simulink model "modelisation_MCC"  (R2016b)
settings: Solver=ode15s  StartTime=0.0  StopTime=25  RelTol=1e-3  EnableMultiTasking=on
undefined symbols (not defined in the file): masse
libraries: fl_lib x13, bibliotheque_pilote x4, nesl_utility x2, elec_lib x1

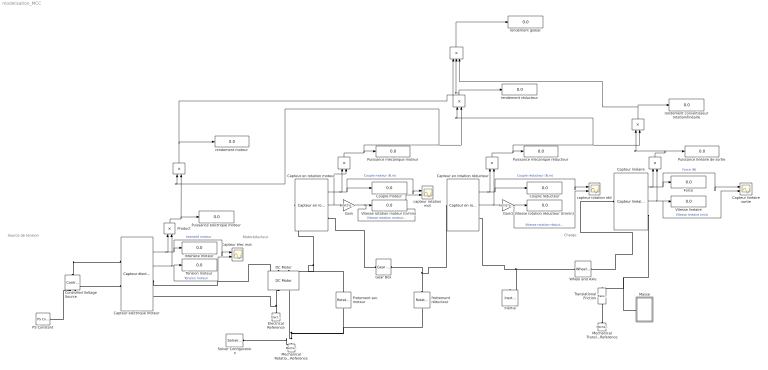
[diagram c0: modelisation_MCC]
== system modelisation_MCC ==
  note: Source de tension
  note: Motoréducteur
  note: Charge
  " " : Product
  " " : Product
  " " : Product
  "                          " : Product  Inputs=*/
  "                           " : Product  Inputs=*/
  "                              " : Product  Inputs=*/
  " " : Product  Inputs=3
  Capteur en rotation moteur : bibliotheque_pilote/Capteur en rotation
  Capteur en rotation réducteur : bibliotheque_pilote/Capteur en rotation
  Capteur linéaire : bibliotheque_pilote/Capteur linéaire
  Capteur linéaire sortie : Scope  NumInputPorts=2
  "Capteur élec mot " : Scope  NumInputPorts=2
  Capteur électrique moteur : bibliotheque_pilote/Capteur électrique
  Controlled Voltage Source : fl_lib/Electrical/Electrical Sources/Controlled Voltage Source
  Couple moteur : Display
  Couple réducteur : Display
  DC Motor : elec_lib/Actuators & Drivers/Rotational Actuators/DC Motor  parameterization=1  Ra=1.27 Ohm  La=0.17 H  emf_or_torque=2  Kv=0.00306 V/rpm  Ki=0.2188 N*m/A  T_stall=219 mN*m  w_max=3920 rpm  w_rated=2670 rpm  P_rated=20 W  V_rated=12 V  J=0.612 g*cm^2  lam_param=2  lam=0 N*m/(rad/s)  i_noload=290 mA  V_i_noload=12 V  speed0=0 rpm  alpha=0.00393 1/K  Tmeas=25 C  thermal_mass=100 J/K  initial_temperature=25 C
  Electrical Reference : fl_lib/Electrical/Electrical Elements/Electrical Reference
  Force : Display
  Frotement sec moteur : fl_lib/Mechanical/Rotational Elements/Rotational Friction  brkwy_trq=0.628 N*m  Col_trq=0.628 N*m  visc_coef=0 N*m/(rad/s)  trans_coef=10 s/rad  vel_thr=1e-04 rad/s  w_specify=off  w_priority=None  w=0 rad/s  t_specify=off  t_priority=None  t=0 N*m
  Gain : Gain  Gain=60/(2*pi)
  Gain1 : Gain  Gain=60/(2*pi)
  Gear Box : fl_lib/Mechanical/Mechanisms/Gear Box  ratio=18  t_in_specify=off  t_in_priority=High  t_in=0 N*m  t_out_specify=off  t_out_priority=High  t_out=0 N*m
  Inertia : fl_lib/Mechanical/Rotational Elements/Inertia  inertia=0.1512 g*cm^2  w_specify=off  w_priority=High  w=0 rad/s  t_specify=off  t_priority=High  t=0 N*m
  Intensité moteur : Display
  Masse : Subsystem
  Mechanical Rotational Reference : fl_lib/Mechanical/Rotational Elements/Mechanical Rotational Reference
  Mechanical Translational Reference : fl_lib/Mechanical/Translational Elements/Mechanical Translational Reference
  PS Constant : fl_lib/Physical Signals/Sources/PS Constant  constant=12
  Product : Product
  Puissance linéaire de sortie : Display
  Puissance mécanique moteur : Display
  Puissance mécanique réducteur : Display
  Puissance électrique moteur : Display
  Solver Configuration : nesl_utility/Solver Configuration  PhysicalDomain=network_engine_domain  SubClassName=solver  LeftPortType=input  RightPortType=generic  Accelerate=off  Tones=[]  Harmonics=[]  SimulateNoise=off  Profile=off  UseLocalSampling=off  EnableSwitchedLinearOptims=on  FrequencyDomain=off  UseCCode=off  RelTol=0.001  AbsTol=1e-06  MinStep=1e-09  ToWorkspace=off  RevertToSquareIcSolve=off  NumHomotopyIterations=100  PhasorMode=off  PhasorModeNumHarmonics=1  OverrideAbsTol=off  DoDC=off  ResidualTolerance=1e-09  UseLocalSolver=off  LocalSolverChoice=NE_BACKWARD_EULER_ADVANCER  LocalSolverSampleTime=0.001  DoFixedCost=off  MaxNonlinIter=3  MaxModeIter=2  LinearAlgebra=Sparse  DelaysMemoryBudget=1024  AutomaticFiltering=on  FilteringTimeConstant=0.001
  Tension moteur : Display
  Translational Friction : fl_lib/Mechanical/Translational Elements/Translational Friction  brkwy_frc=70 N  Col_frc=70 N  visc_coef=0 N/(m/s)  trans_coef=10 s/m  vel_thr=1e-4 m/s  v_specify=off  v_priority=High  v=0 m/s  f_specify=off  f_priority=High  f=0 N
  Vitesse linéaire : Display
  Vitesse rotation moteur (tr/min) : Display
  Vitesse rotation réducteur (tr/min) : Display
  Wheel and Axle : fl_lib/Mechanical/Mechanisms/Wheel and Axle  R=7.5 mm  or=1  t_specify=off  t_priority=High  t=0 N*m  f_specify=off  f_priority=High  f=0 N
  capteur rotation mot : Scope  NumInputPorts=2
  capteur rotation réd : Scope  NumInputPorts=2
  frottement réducteur : fl_lib/Mechanical/Rotational Elements/Rotational Friction  brkwy_trq=43 mN*m  Col_trq=43 mN*m  visc_coef=0 N*m/(rad/s)  trans_coef=10 s/rad  vel_thr=1e-4 rad/s  w_specify=off  w_priority=High  w=0 rad/s  t_specify=off  t_priority=High  t=0 N*m
  rendement convertisseur rotation/linéaire : Display
  rendement global : Display
  rendement moteur : Display
  rendement réducteur : Display
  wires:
  Capteur électrique moteur/1 -> Product/1, "Capteur élec mot "/1, Intensité moteur/1  "Intensité moteur"
  Product/1 -> Puissance électrique moteur/1, "                              "/2
  Capteur électrique moteur/2 -> Product/2, "Capteur élec mot "/2, Tension moteur/1  "Tension moteur"
  Capteur en rotation moteur/2 -> Gain/1, " "/2
  Capteur en rotation moteur/1 -> " "/1, capteur rotation mot/1, Couple moteur/1  "Couple moteur (N.m)"
  " "/1 -> "                              "/1, "                          "/2, Puissance mécanique moteur/1
  Capteur en rotation réducteur/2 -> Gain1/1, " "/2
  Capteur en rotation réducteur/1 -> " "/1, capteur rotation réd/1, Couple réducteur/1  "Couple réducteur (N.m)"
  " "/1 -> "                          "/1, "                           "/2, Puissance mécanique réducteur/1
  Capteur linéaire/1 -> " "/1, Capteur linéaire sortie/1, Force/1  "Force (N)"
  Capteur linéaire/2 -> " "/2, Capteur linéaire sortie/2, Vitesse linéaire/1  "Vitesse linéaire (m/s)"
  " "/1 -> "                           "/1, Puissance linéaire de sortie/1
  "                           "/1 -> rendement convertisseur rotation/linéaire/1, " "/3
  "                          "/1 -> " "/2, rendement réducteur/1
  "                              "/1 -> " "/1, rendement moteur/1
  " "/1 -> rendement global/1
  Gain/1 -> capteur rotation mot/2, Vitesse rotation moteur (tr/min)/1  "Vitesse rotation moteur (tr/min)"
  Gain1/1 -> Vitesse rotation réducteur (tr/min)/1, capteur rotation réd/2  "Vitesse rotation réducteur (tr/min)"
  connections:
  Solver Configuration/RConn1 -- frottement réducteur/RConn1 -- Frotement sec moteur/RConn1 -- DC Motor/RConn2 -- Mechanical Rotational Reference/LConn1
  Electrical Reference/LConn1 -- DC Motor/RConn1 -- Capteur électrique moteur/RConn2
  PS Constant/RConn1 -- Controlled Voltage Source/RConn1
  Wheel and Axle/LConn1 -- Capteur en rotation réducteur/RConn1 -- Inertia/LConn1
  Mechanical Translational Reference/LConn1 -- Translational Friction/RConn1
  Controlled Voltage Source/LConn1 -- Capteur électrique moteur/LConn1
  Controlled Voltage Source/RConn2 -- Capteur électrique moteur/LConn2
  Capteur électrique moteur/RConn1 -- DC Motor/LConn1
  frottement réducteur/LConn1 -- Capteur en rotation réducteur/LConn1 -- Gear Box/RConn1
  Capteur linéaire/LConn1 -- Wheel and Axle/RConn1
  Capteur en rotation moteur/LConn1 -- Frotement sec moteur/LConn1 -- DC Motor/LConn2
  Capteur en rotation moteur/RConn1 -- Gear Box/LConn1
  Capteur linéaire/RConn1 -- Masse/LConn1 -- Translational Friction/LConn1

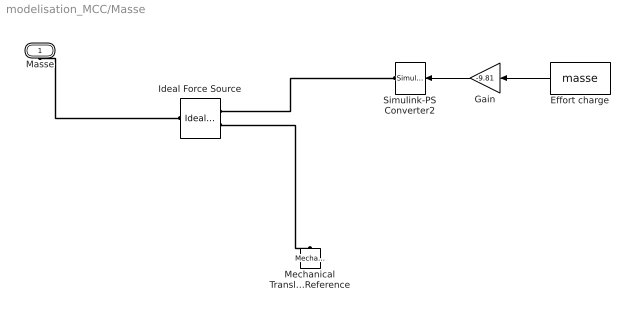
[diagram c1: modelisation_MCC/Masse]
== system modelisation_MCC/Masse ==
  Effort charge : Constant  Value=masse
  Gain : Gain  Gain=-9.81
  Ideal Force Source : fl_lib/Mechanical/Mechanical Sources/Ideal Force Source
  Mechanical Translational Reference : fl_lib/Mechanical/Translational Elements/Mechanical Translational Reference
  Simulink-PS Converter2 : nesl_utility/Simulink-PS Converter  PhysicalDomain=network_engine_domain  SubClassName=ps_input  LeftPortType=input  RightPortType=output  PseudoPeriodic=off  Frequencies=[]  NoiseDistribution=none  NoiseParameters=[]  Unit=N  AffineConversion=off  InputFiltering=off  SimscapeFilterOrder=1  InputFilterTimeConstant=.001  UdotUserProvided=0
  Masse : PMIOPort  Port=1  Side=Left
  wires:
  Effort charge/1 -> Gain/1
  Gain/1 -> Simulink-PS Converter2/1
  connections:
  Ideal Force Source/RConn2 -- Mechanical Translational Reference/LConn1
  Ideal Force Source/RConn1 -- Simulink-PS Converter2/RConn1
  Ideal Force Source/LConn1 -- Masse/RConn1
